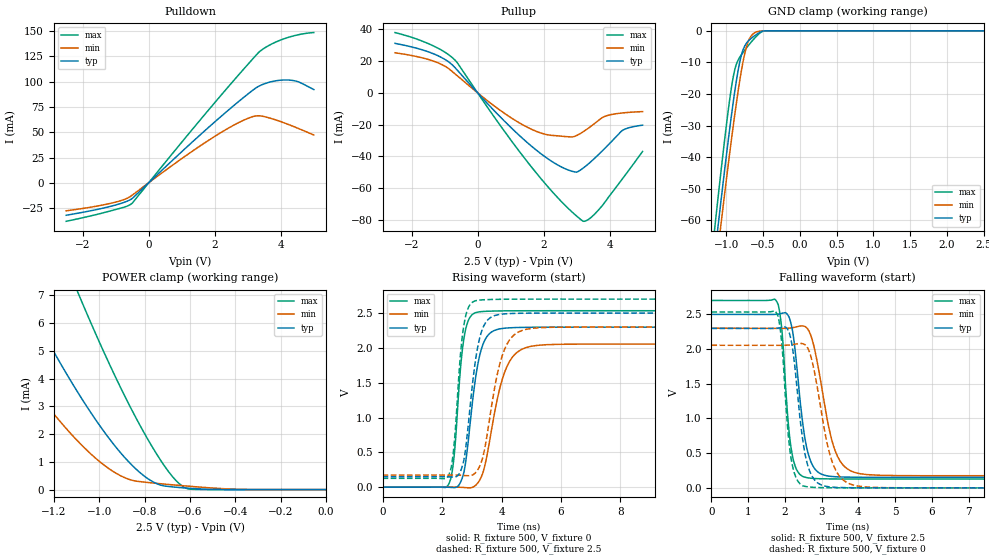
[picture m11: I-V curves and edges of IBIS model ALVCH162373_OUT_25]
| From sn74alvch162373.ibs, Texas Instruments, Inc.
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[Model]   ALVCH162373_OUT_25
Model_type  3-state
Enable   Active-Low
Vref =   0
Rref =   500
Cref =   30p
Vmeas =   1.25
| variable   typ   min   max
C_comp   7.02pF   6.01pF   8.37pF
| C_pullup   5.48pF   4.02pF   8.53pF
| C_pulldown   4.51pF   3.74pF   5.78pF
| C_tri-state   7.02pF   6.01pF   8.37pF
[Temperature Range]   40   100   -40
| Ambient temperature   25   85   -40
[Voltage range]   2.5   2.3   2.7
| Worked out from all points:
|   slope of the pulldown table from 0 to 0.375 V, typ, clamps not added: 32.2 ohm
|   slope of the pullup table from 0 to 0.375 V, typ, clamps not added: 44.5 ohm
|   GND clamp passes 1 mA (typ) near -0.58 V on its own axis
|   POWER clamp passes 1 mA (typ) near -0.87 V on its own axis
|   rising waveform, R_fixture 500, V_fixture 0: 20-80 % time 413ps typ, 609ps min, 280ps max; typ from 0 V to 2.3 V
|   falling waveform, R_fixture 500, V_fixture 2.5: 20-80 % time 310ps typ, 470ps min, 218ps max; typ from 2.5 V to 0.151 V
|   rising waveform, R_fixture 500, V_fixture 2.5: 20-80 % time 396ps typ, 559ps min, 276ps max; typ from 0.151 V to 2.5 V
|   falling waveform, R_fixture 500, V_fixture 0: 20-80 % time 308ps typ, 450ps min, 222ps max; typ from 2.3 V to 0 V
[GND Clamp]
| ALVCH162373_OUT_25
|   Voltage   I(typ)   I(min)   I(max)
-2.5V     -365.5mA   -364.1mA   -369.1mA
-1.15V    -70.09mA   -77.1mA    -61.39mA
-1.1V     -59.88mA   -67.15mA   -50.77mA
-1.07V    -53.84mA   -61.25mA   -44.52mA
-920mV    -25.39mA   -33.03mA   -16.8mA
-875mV    -17.97mA   -25.23mA   -11.65mA
-820mV    -10.46mA   -16.49mA   -8.56mA
-775mV    -6.349mA   -10.35mA   -7.012mA
-720mV    -3.805mA   -4.788mA   -5.315mA
-605mV    -1.421mA   -519.8uA   -2.128mA
-475mV    -16.57uA   -54.22uA   -12.1uA
2.5V      83.81pA    43.75nA    39.19pA
[POWER Clamp]
| ALVCH162373_OUT_25
|   Voltage   I(typ)   I(min)   I(max)
-2.5V     28.66mA    20.76mA    40.74mA
-1.575V   10.98mA    7.111mA    17.51mA
-1.55V    10.55mA    6.788mA    16.93mA
-1.33V    6.926mA    4.117mA    11.98mA
-1.205V   5.038mA    2.778mA    9.335mA
-1.085V   3.383mA    1.667mA    6.931mA
-950mV    1.776mA    714.5uA    4.435mA
-835mV    718.9uA    302.8uA    2.539mA
-740mV    193.1uA    219.7uA    1.192mA
-640mV    70.19uA    146.2uA    164.5uA
-575mV    31.48uA    102.2uA    6.344uA
-31.15fV  83.81pA    322.9pA    46.7pA
[Pulldown]
| ALVCH162373_OUT_25
|   Voltage   I(typ)   I(min)   I(max)
-2.5V     -32.17mA   -27.74mA   -38.14mA
-1.125V   -23.09mA   -20.14mA   -27.56mA
-730mV    -19.19mA   -16.41mA   -24.02mA
-510mV    -15.79mA   -12.5mA    -20.47mA
1.78V     53.88mA    41.29mA    70.78mA
2.595V    76.92mA    57.38mA    102mA
3.145V    91.41mA    65.4mA     122.4mA
3.335V    95.53mA    66.27mA    129.1mA
3.51V     98.04mA    65.4mA     133.4mA
4.13V     101.8mA    58.95mA    142.9mA
4.52V     100mA      53.93mA    146.4mA
5V        92.27mA    47.27mA    148.7mA
[Pullup]
| ALVCH162373_OUT_25
|   Voltage   I(typ)   I(min)   I(max)
-2.5V     31.01mA    25.1mA     37.8mA
-1.325V   24.4mA     19.8mA     29.3mA
-685mV    15.82mA    11.91mA    20.57mA
660mV     -14.56mA   -10.62mA   -19.69mA
1.65V     -33.8mA    -23.08mA   -47.03mA
2.67V     -47.85mA   -27.51mA   -71.03mA
2.99V     -49.83mA   -26.97mA   -77.22mA
3.19V     -47.49mA   -24.63mA   -80.57mA
3.605V    -40.02mA   -18.35mA   -74.96mA
3.885V    -34.32mA   -14.62mA   -68mA
4.38V     -23.78mA   -12.7mA    -54.32mA
5V        -20.36mA   -11.83mA   -36.84mA
[Ramp]
| ALVCH162373_OUT_25
| variable   typ   min   max
dV/dt_r   1.38/4.17E-10   1.24/6.17E-10   1.52/2.90E-10
dV/dt_f   1.42/3.18E-10   1.29/4.79E-10   1.56/2.27E-10
R_load = 500
[Rising Waveform]
| ALVCH162373_OUT_25
R_fixture =   500
C_fixture =   0
L_fixture =   0
V_fixture =   0
V_fixture_min = 0
V_fixture_max = 0
|   Time   V(typ)   V(min)   V(max)
0s        318.3pV    1.281nV    228.9pV
2.21ns    -1.178mV   934.2uV    32.36mV
2.4ns     -7.298mV   882.3uV    425.8mV
2.615ns   66.57mV    -1.569mV   1.684V
2.75ns    248.7mV    -5.202mV   2.172V
3.185ns   1.725V     52.49mV    2.512V
3.505ns   2.16V      442.4mV    2.525V
4.12ns    2.283V     1.668V     2.532V
4.97ns    2.296V     2.02V      2.533V
24.99ns   2.297V     2.055V     2.533V
[Falling Waveform]
| ALVCH162373_OUT_25
R_fixture =   500
C_fixture =   0
L_fixture =   0
V_fixture =   2.5
V_fixture_min = 2.3
V_fixture_max = 2.7
|   Time   V(typ)   V(min)   V(max)
0s        2.5V       2.3V       2.7V
1.785ns   2.502V     2.298V     2.677V
1.915ns   2.515V     2.298V     2.288V
2.07ns    2.497V     2.3V       1.067V
2.175ns   2.345V     2.305V     551.7mV
2.6ns     562.6mV    2.301V     147.3mV
2.87ns    241.1mV    1.838V     133.1mV
3.365ns   160.6mV    537.7mV    128.5mV
4.03ns    152.7mV    205.2mV    127.4mV
24.99ns   150.8mV    173.8mV    127mV
[Rising Waveform]
| ALVCH162373_OUT_25
R_fixture =   500
C_fixture =   0
L_fixture =   0
V_fixture =   2.5
V_fixture_min = 2.3
V_fixture_max = 2.7
|   Time   V(typ)   V(min)   V(max)
0s        150.8mV    173.8mV    127mV
2.21ns    149mV      174.1mV    161.5mV
2.39ns    143.7mV    173.8mV    551mV
2.6ns     211.2mV    171.2mV    1.811V
2.72ns    364mV      168.4mV    2.292V
3.125ns   1.825V     207.9mV    2.677V
3.45ns    2.352V     590.3mV    2.692V
4.04ns    2.486V     1.91V      2.698V
4.82ns    2.498V     2.266V     2.7V
24.99ns   2.5V       2.3V       2.7V
[Falling Waveform]
| ALVCH162373_OUT_25
R_fixture =   500
C_fixture =   0
L_fixture =   0
V_fixture =   0
V_fixture_min = 0
V_fixture_max = 0
|   Time   V(typ)   V(min)   V(max)
0s        2.297V     2.055V     2.533V
1.78ns    2.3V       2.054V     2.511V
1.91ns    2.311V     2.054V     2.109V
2.075ns   2.282V     2.057V     855.1mV
2.17ns    2.123V     2.062V     417.7mV
2.56ns    455.4mV    2.056V     19.98mV
2.815ns   108.7mV    1.64V      6.179mV
3.3ns     10.1mV     353.9mV    1.396mV
3.98ns    1.452mV    26.43mV    271.6uV
24.99ns   -2.06nV    -2.326nV   4.803nV
